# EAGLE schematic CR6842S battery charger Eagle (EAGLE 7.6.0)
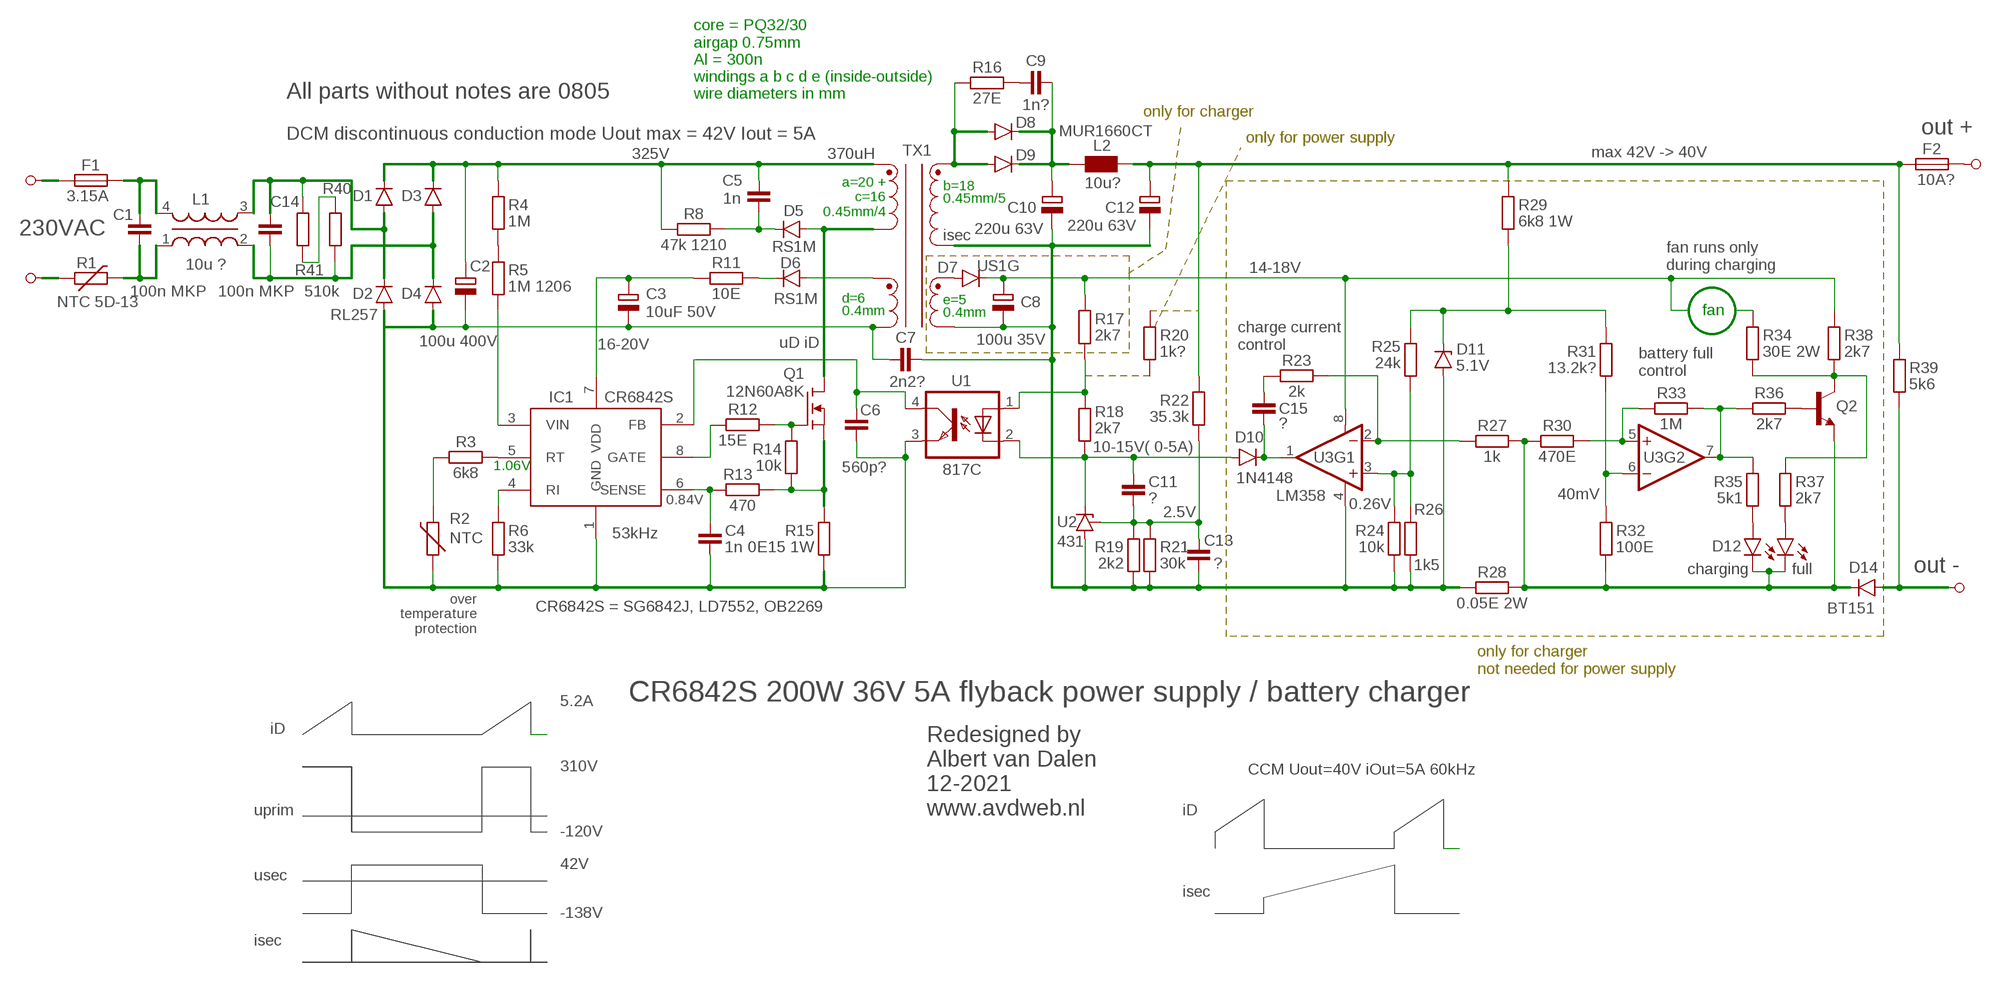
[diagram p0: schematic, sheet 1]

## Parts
C1  100n MKP  SMD-C-0603-SMALL  [0603-SMALL]
C2  100u 400V  CAP-POL""  [E3,5-8]
C3  10uF 50V  CAP-POL""  [E3,5-8]
C4  1n  SMD-C-0603-SMALL  [0603-SMALL]
C5  1n  SMD-C-0603-SMALL  [0603-SMALL]
C6  560p?  SMD-C-0603-SMALL  [0603-SMALL]
C7  2n2?  SMD-C-0603-SMALL  [0603-SMALL]
C8  100u 35V  CAP-POL""  [E3,5-8]
C9  1n?  SMD-C-0603-SMALL  [0603-SMALL]
C10  220u 63V  CAP-POL""  [E3,5-8]
C11  ?  SMD-C-0603-SMALL  [0603-SMALL]
C12  220u 63V  CAP-POL""  [E3,5-8]
C13  ?  SMD-C-0603-SMALL  [0603-SMALL]
C14  100n MKP  SMD-C-0603-SMALL  [0603-SMALL]
C15  ?  SMD-C-0603-SMALL  [0603-SMALL]
D1  RL257  DIODEPTH  [DIODE-1N4001]
D2  RL257  DIODEPTH  [DIODE-1N4001]
D3  RL257  DIODEPTH  [DIODE-1N4001]
D4  RL257  DIODEPTH  [DIODE-1N4001]
D5  RS1M  DIODE-SMDSMA  [SMA]
D6  RS1M  DIODE-SMDSMA  [SMA]
D7  US1G  DIODE-SMDSMA  [SMA]
D8  MUR1660CT  DIODE-SMDSMA  [SMA]
D9  MUR2007CT  DIODE-SMDSMA  [SMA]
D10  1N4148  DIODE-SMD  [SOD-323]
D11  5.1V  ZENER  [SOD-323]
D12  green  LED  [LED-0603]
D13  red?????  LED  [LED-0603]
D14  BT151  DIODE-SMD  [SOD-323]
F1  3.15A  FUSE  [1206]
F2  10A?  FUSE  [1206]
IC1  CR6842S  SG6842JLSZ  [SOIC127P599X175-8N]
J1  230VAC  PIN  [PIN]
J2  230VAC  PIN  [PIN]
J3  out -  PIN  [PIN]
J4  out +  PIN  [PIN]
L1  10u ?  COMMON_MODE_INDUCTOR"  [1X04]
L2  10u?  INDUCTOR-SMD'  [0805-CAP]
Q1  12N60A8K  MOSFET-N-CHTO-220V  [TO220V]
Q2  TRANSISTOR_NPN2N3904  [TO-92]
R1  NTC 5D-13  PTC  [1206]
R2  NTC  PTC  [1206]
R3  6k8  SMD-R-0603-SMALL  [0603-SMALL]
R4  1M  SMD-R-0603-SMALL  [0603-SMALL]
R5  1M 1206  SMD-R-0603-SMALL  [0603-SMALL]
R6  33k  SMD-R-0603-SMALL  [0603-SMALL]
R8  47k 1210  SMD-R-0603-SMALL  [0603-SMALL]
R11  10E  SMD-R-0603-SMALL  [0603-SMALL]
R12  15E  SMD-R-0603-SMALL  [0603-SMALL]
R13  470  SMD-R-0603-SMALL  [0603-SMALL]
R14  10k  SMD-R-0603-SMALL  [0603-SMALL]
R15  0E15 1W  SMD-R-0603-SMALL  [0603-SMALL]
R16  27E  SMD-R-0603-SMALL  [0603-SMALL]
R17  2k7  SMD-R-0603-SMALL  [0603-SMALL]
R18  2k7  SMD-R-0603-SMALL  [0603-SMALL]
R19  2k2  SMD-R-0603-SMALL  [0603-SMALL]
R20  1k?  SMD-R-0603-SMALL  [0603-SMALL]
R21  30k  SMD-R-0603-SMALL  [0603-SMALL]
R22  35.3k  SMD-R-0603-SMALL  [0603-SMALL]
R23  2k  SMD-R-0603-SMALL  [0603-SMALL]
R24  10k  SMD-R-0603-SMALL  [0603-SMALL]
R25  24k  SMD-R-0603-SMALL  [0603-SMALL]
R26  1k5  SMD-R-0603-SMALL  [0603-SMALL]
R27  1k  SMD-R-0603-SMALL  [0603-SMALL]
R28  0.05E 2W  SMD-R-0603-SMALL  [0603-SMALL]
R29  6k8 1W  SMD-R-0603-SMALL  [0603-SMALL]
R30  470E  SMD-R-0603-SMALL  [0603-SMALL]
R31  13.2k?  SMD-R-0603-SMALL  [0603-SMALL]
R32  100E  SMD-R-0603-SMALL  [0603-SMALL]
R33  1M  SMD-R-0603-SMALL  [0603-SMALL]
R34  30E 2W  SMD-R-0603-SMALL  [0603-SMALL]
R35  5k1  SMD-R-0603-SMALL  [0603-SMALL]
R36  2k7  SMD-R-0603-SMALL  [0603-SMALL]
R37  2k7  SMD-R-0603-SMALL  [0603-SMALL]
R38  2k7  SMD-R-0603-SMALL  [0603-SMALL]
R39  5k6  SMD-R-0603-SMALL  [0603-SMALL]
R40  510k  SMD-R-0603-SMALL  [0603-SMALL]
R41  510k  SMD-R-0603-SMALL  [0603-SMALL]
TX1  TRANSFORMER-CHARGER-CR6842S"  [1X08]
U1  817C  LTV816  [DIL04]
U2  431  431'  [1X03]
U3  LM358  [DIP08]

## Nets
2.5V: C11.2 C13.1 R19.2 R21.2 R22.1 U2.3
14-18V: C8.+ D7.C R17.2 R38.2 U3.8(V+)
16-20V: C3.+ IC1.7(VDD) R11.1
36V: C12.+ F2.1 L2.2 R22.2 R29.2 R39.2
325V: C2.+ C5.1 D1.C D3.C R4.2 R8.1 TX1.4
N$1: R2.2 R3.1
N$2: IC1.3(VIN) R5.1
N$3: IC1.8(GATE) R12.1
N$4: C4.1 IC1.6(SENSE) R13.1
N$5: Q1.3(S) R13.2 R14.1 R15.2
N$6: Q1.1(G) R12.2 R14.2
N$7: IC1.5(RT) R3.2
N$9: IC1.4(RI) R6.2
N$10: R4.1 R5.2
N$11: R34.2
N$12: C2.- C3.- C4.2 C6.2 C7.1 D2.A D4.A IC1.1(GND) R2.1 R6.1 R15.1 TX1.1 U1.3(EMIT)
N$13: D6.A TX1.2
N$14: D5.A Q1.2(D) TX1.3
N$15: D6.C R11.2
N$16: C5.2 D5.C R8.2
N$20: C7.2 C8.- C10.- C12.- C13.2 D11.A R19.1 R21.1 R24.1 R26.1 R28.1 TX1.6 TX1.7 U2.1(A) U3.4(V-)
N$21: C14.2 D3.A D4.C L1.2 R40.1
N$22: C1.1 F1.2 L1.4
N$23: C1.2 L1.1 R1.2
N$24: F1.1 J1.1
N$25: J2.1 R1.1
N$26: R17.1 R18.2 U1.1(A)
N$28: C11.1 D10.A R18.1 U1.2(C) U2.2(C)
N$29: C15.1 R23.1
N$30: D7.A TX1.5
N$31: R40.2 R41.1
N$32: D8.A D9.A R16.1 TX1.8
N$33: C9.2 C10.+ D8.C D9.C L2.1
N$34: C9.1 R16.2
N$35: R31.1 R32.2 U3.6(-IN)
N$36: C14.1 D1.A D2.C L1.3 R41.2
N$37: R30.2 R33.1 U3.5(+IN)
N$38: C15.2 D10.C U3.1(OUT)
N$40: R23.2 R27.1 U3.2(-IN)
N$41: R24.2 R25.1 R26.2 U3.3(+IN)
N$42: R33.2 R35.2 R36.1 U3.7(OUT)
N$43: D12.A R35.1
N$44: D11.C R25.2 R29.1 R31.2
N$45: D14.A J3.1 R39.1
N$46: F2.2 J4.1
N$47: Q2.2(B) R36.2
N$48: Q2.3(C) R34.1 R37.2 R38.1
N$49: D13.A R37.1
N$50: D12.C D13.C D14.C Q2.1(E) R27.2 R28.2 R30.1 R32.1
N$51: C6.1 IC1.2(FB) U1.4(COL)
Unconnected: R20.1 R20.2

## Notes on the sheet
- All parts without notes are 0805
- core = PQ32/30
  airgap 0.75mm
  Al = 300n
  windings a b c d e (inside-outside)
  wire diameters in mm
- only for charger
- DCM discontinuous conduction mode Uout max = 42V Iout = 5A | only for power supply
- 370uH | max 42V -> 40V
- a=20 +
  c=16
  0.45mm/4
- b=18
  0.45mm/5
- isec
- fan runs only 
  during charging
- d=6
  0.4mm
- fan
- e=5
  0.4mm
- uD iD
- charge current 
  control
- battery full 
  control
- 10-15V( 0-5A)
- 1.06V
- 40mV
- 0.26V
- 0.84V
- 53kHz
- charging | full
- over
  temperature
  protection
- CR6842S = SG6842J, LD7552, OB2269
- only for charger
  not needed for power supply
- CR6842S 200W 36V 5A flyback power supply / battery charger
- 5.2A
- iD
- 310V | CCM Uout=40V iOut=5A 60kHz
- uprim
- Redesigned by
  Albert van Dalen
  12-2021
  www.avdweb.nl
- iD
- -120V
- 42V
- usec
- isec
- -138V
- isec

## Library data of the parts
C1 C4-C7 C9 C11 C13-C15 = Albert:SMD-C: Capacitors
C2 C3 C8 C10 C12 = Albert:CAP-POL
D1-D4 = SparkFun-DiscreteSemi:DIODE: Diode
D5-D10 D14 = Albert:DIODE-SMD
D11 = Albert:ZENER
D12 D13 = Albert:LED
F1 F2 = Albert:FUSE; VALUE: 5A
IC1 = SamacSys_Parts:SG6842JLSZ: Highly-Integrated Green-Mode PWM Controller Source: Datasheet; DESCRIPTION: Highly-Integrated Green-Mode PWM Controller; HEIGHT: 1.752mm; MANUFACTURER_NAME: ON Semiconductor; MANUFACTURER_PART_NUMBER: SG6842JLSZ; MOUSER_PART_NUMBER: N/A; MOUSER_PRICE-STOCK: https://www.mouser.co.uk/ProductDetail/ON-Semiconductor-Fairchild/SG6842JLSZ?qs=C5IC29ode6usIsNMjYwZZQ%3D%3D
J1-J4 = Albert:PIN: PIN HEADER
L1 = Albert:COMMON_MODE_INDUCTOR: Small transformers
L2 = Albert:INDUCTOR-SMD
Q1 = Albert:MOSFET-N-CH
Q2 = SparkFun-DiscreteSemi:TRANSISTOR_NPN: Generic NPN BJT MMBT2222A - TRANS-08049 (SOT-23, 1A 40V) MPSA42 - TRANS-09116 (SOT-23, 500mA 300V) MMBT5088LT1G - TRANS-11160 (SOT-23, 50 mA 30V) BC547 - COM-08928 (TO-92 45V 100mA) (1.Collector 2.Base 3.Emitter) 2N3904 - COM-00521 (TO-92 40V 200mA) (1.Emitter 2.Base 3.Collector) P2N2222A -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; PROD_ID: TRANS-08447
R1 R2 = Albert:PTC; VALUE: 5A
R3-R6 R8 R11-R41 = Albert:SMD-R: Resistors
TX1 = Albert:TRANSFORMER-CHARGER-CR6842S: Transformer with 4 independent windings
U1 = Albert:LTV816: OPTO COUPLER Source: LITEON, LTV816.pdf; OC_FARNELL: unknown; OC_NEWARK: unknown
U2 = Albert:431
U3 = SparkFun-AnalogIC:LM358: Jellybean op-amp; PROD_ID: IC-09172

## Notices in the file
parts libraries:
SparkFun-DiscreteSemi: Licensing: Creative Commons ShareAlike 4.0 International - https://creativecommons.org/licenses/by-sa/4.0
